|   Microchip Technology Inc.
|   PolarFire IBIS Model
[IBIS ver]   5.0
[File name]   polarfire_hsio_diff.ibs
[File Rev]   2.3
[Date]   Wed Nov 22 2023
[Source] Simulated Models ONLY.
   All data is based on Spice simulation. All performed at Microchip Technology Inc.
[Notes]   This IBIS file is for HSIO Differential standards.
   Please refer to polarfire_hsio_se.ibs for HSIO single ended Standards Configurations,
   and refer to polarfire_gpio_se.ibs and polarfire_gpio_diff.ibs for GPIO Configurations.
   The package parasitics of various package types are given.
   Uncomment the appropriate package before simulations.
   Revision History
   Rev 2.3: 22-Nov-2023
   - Added mixed mode receiver support:
   - Input buffers: HSTL12_18_ODT-OFF,HSTL12_15_ODT-OFF,HSTL12_135_ODT-OFF,
   HSTL135_18_ODT-OFF,HSTL135_15_ODT-OFF,HSTL15_18_ODT-OFF,
   HSUL12_18_ODT-OFF,HSUL12_18_ODT-60,HSUL12_18_ODT-120,HSUL12_18_ODT-240,
   HSUL12_15_ODT-OFF,HSUL12_15_ODT-60,HSUL12_15_ODT-120,HSUL12_15_ODT-240,
   HSUL12_135_ODT-OFF,HSUL12_135_ODT-60,HSUL12_135_ODT-120,HSUL12_135_ODT-240,
   POD12_18_ODT-OFF,POD12_15_ODT-OFF,POD12_135_ODT-OFF,SSTL135_18_ODT-OFF,
   SSTL135_15_ODT-OFF,SSTL15_18_ODT-OFF
   Rev 2.2: 20-Jun-2023
   - Added VCM-LOW configuration support for LVDS18,RSDS18,MINILVDS18,
   SUBLVDS18,PPDS18,SLVS18,HCSL18 receivers
   - Updated Vinl and Vinh values of LVDS18,SLVS18 receivers
   Rev 2.1: 14-Sep-2022
   - Added MPF050 device with RLC package data in [Package] section
   - Added LPDDR4 LVSTL11D I/O standard
   - Added RLC package type of FCG784N for MPF300T/TS device
   - Update RLC values of 200T-FCVG484 device package data
[Disclaimer] This information is for board design considerations.
   Simulation based V/I curves contained in this model file are
   considered preliminary until verified against bench
   measurements. Maximum currents may vary from part to part but
   should not exceed maximum I/V curves provided in this model file.
[Copyright]  (c) 2023, Microchip Technology Inc., All Rights Reserved.
| ADDITIONAL NOTES
| Warnings for ISSO Pullup, Pulldown currents being non-zero are expected.
| The naming conventions used in the signal_name/model_name are as follows:
| SLEW-#  - Slew setting,OFF or ON represented by #
| HYST-# and HYS-#  - Hysteresis setting,OFF or ON represented by #
| #mA   - Driver current strength, value represented by #
| #ohm   - Driver impedance mode, value represented by #
| ODT-# and OD-#   - Series on-die termination, impedance value represented by #
| C1   - Refers to Class-I driver models
| C2   - Refers to Class-II driver models
| #_I   - Refers to input models ,  model name represented by #
| #_O   - Refers to output models , model name represented by #
| VCML   - Refers to LOW Vcm setting
| VCMM   - Refers to MID Vcm setting
| IBIS MODEL CHECKLIST
| Microchip Technology Inc. is dedicated to releasing quality IBIS models to customers.
| The following items have been
| verified for this IBIS model before release:
| 1)  Checked IBIS model by the golden parser ibischk5 [Complete]
| 2)  Ensured no errors reported by golden parser
|   for the IBIS model [Complete]
| 3)  Defined Vinl and Vinh for receivers [Complete]
| 4)  Defined Standard Load and Vmeas values for drivers [Complete]
| 5)  Defined overshoots for drivers and receivers [NA]
| 6)  Validated Ramp Values[]
| 7)  Defined V-T Tables for all output drivers [Complete]
| 8)  Validated [Diff Pins] [Complete]
| 9)  Verified Package Parasitics [Complete]
| 10) Defined Standard Load Parameters and Specifications
|   for waveforms [Complete]
| 11) Defined and Validate Pin mappings [Complete]
| 12) Verified C_comp_pullup and C_comp_pulldown Values []
| 13) Visually Inspected I-V Curves and V-T Tables  [Complete]
| 14) Presented Typ/Min/Max Values in the correct order for
|   all tables and parameters [Complete]
| 15) Simulated all output models with standard load and
|   switching through Vmeas [Complete]
| 16) Simulated all receiver models  [Complete]
| 17) Validated Models selectors. [NA]
| 18) Visually inspected Spice and IBIS correlation for
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[Component]   PolarFire
[Manufacturer]   Microchip Technology Inc.
[Package]
|   typ   min   max
|MPF050T/TL/TLS/TS
|R_pkg   0.424   NA   NA   | MPF050T/TL/TLS/TS-FCSG325
|L_pkg   2.847nH   NA   NA   | MPF050T/TL/TLS/TS-FCSG325
|C_pkg   1.075pF   NA   NA   | MPF050T/TL/TLS/TS-FCSG325
|R_pkg   0.726   NA   NA   | MPF050T/TL/TLS/TS-FCVG484
|L_pkg   5.270nH   NA   NA   | MPF050T/TL/TLS/TS-FCVG484
|C_pkg   1.827pF   NA   NA   | MPF050T/TL/TLS/TS-FCVG484
|MPF100T/TL/TLS/TS
|R_pkg   0.300925   NA   NA   | MPF100T/TL/TLS/TS-FCSG325
|L_pkg   2.47653nH   NA   NA   | MPF100T/TL/TLS/TS-FCSG325
|C_pkg   1.00755pF   NA   NA   | MPF100T/TL/TLS/TS-FCSG325
|R_pkg   0.873007   NA   NA   | MPF100T/TL/TLS/TS-FCG484
|L_pkg   5.7244nH   NA   NA   | MPF100T/TL/TLS/TS-FCG484
|C_pkg   2.04208pF   NA   NA   | MPF100T/TL/TLS/TS-FCG484
|R_pkg   0.61   NA   NA   | MPF100T/TL/TLS/TS-FCVG484
|L_pkg   4.49536nH   NA   NA   | MPF100T/TL/TLS/TS-FCVG484
|C_pkg   1.77743pF   NA   NA   | MPF100T/TL/TLS/TS-FCVG484
|MPF200T/TL/TLS/TS
|R_pkg   0.570552   NA   NA   | MPF200T/TL/TLS/TS-FCSG325
|L_pkg   4.57321nH   NA   NA   | MPF200T/TL/TLS/TS-FCSG325
|C_pkg   1.39793pF   NA   NA   | MPF200T/TL/TLS/TS-FCSG325
|R_pkg   0.813737   NA   NA   | MPF200T/TL/TLS/TS-FCG484
|L_pkg   5.39433nH   NA   NA   | MPF200T/TL/TLS/TS-FCG484
|C_pkg   1.90867pF   NA   NA   | MPF200T/TL/TLS/TS-FCG484
|R_pkg   0.592554   NA   NA   | MPF200T/TL/TLS/TS-FCVG484
|L_pkg   4.00867nH   NA   NA   | MPF200T/TL/TLS/TS-FCVG484
|C_pkg   1.56354pF   NA   NA   | MPF200T/TL/TLS/TS-FCVG484
|R_pkg   0.39999   NA   NA   | MPF200T/TL/TLS/TS-FCSG536
|L_pkg   3.20603nH   NA   NA   | MPF200T/TL/TLS/TS-FCSG536
|C_pkg   1.22995pF   NA   NA   | MPF200T/TL/TLS/TS-FCSG536
|R_pkg   1.32073   NA   NA   | MPF200T/TL/TLS/TS-FCG784
|L_pkg   8.15293nH   NA   NA   | MPF200T/TL/TLS/TS-FCG784
|C_pkg   2.72193pF   NA   NA   | MPF200T/TL/TLS/TS-FCG784
|MPF300T/TL/TLS/TS
|R_pkg   0.713491   NA   NA   | MPF300T/TL/TLS/TS-FCG484
|L_pkg   4.77635nH   NA   NA   | MPF300T/TL/TLS/TS-FCG484
|C_pkg   1.82577pF   NA   NA   | MPF300T/TL/TLS/TS-FCG484
|R_pkg   0.493927   NA   NA   | MPF300T/TL/TLS/TS-FCVG484
|L_pkg   3.29806nH   NA   NA   | MPF300T/TL/TLS/TS-FCVG484
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R_pkg   1.65645   NA   NA   | MPF300T/TL/TLS/TS-FCG1152
L_pkg   9.92288nH   NA   NA   | MPF300T/TL/TLS/TS-FCG1152
C_pkg   3.06321pF   NA   NA   | MPF300T/TL/TLS/TS-FCG1152
|MPF500T/TL/TLS/TS
|R_pkg   0.914871   NA   NA   | MPF500T/TL/TLS/TS-FCG784
|L_pkg   5.88658nH   NA   NA   | MPF500T/TL/TLS/TS-FCG784
|C_pkg   2.0993pF   NA   NA   | MPF500T/TL/TLS/TS-FCG784
|R_pkg   1.46382   NA   NA   | MPF500T/TL/TLS/TS-FCG1152
|L_pkg   9.31721nH   NA   NA   | MPF500T/TL/TLS/TS-FCG1152
|C_pkg   2.98723pF   NA   NA   | MPF500T/TL/TLS/TS-FCG1152
| End Header
| The PIN numbers given below are examples. They do not correspond to
| device pin numbers.
[Pin]   signal_name   model_name   R_pin   L_pin   C_pin
1N   SSTL18D_C1_60ohm_SLEW-OFF_N_O   SSTL18_C1_60ohm_SLEW-OFF_HSIO_O
1P   SSTL18D_C1_60ohm_SLEW-OFF_P_O   SSTL18_C1_60ohm_SLEW-OFF_HSIO_O
2N   SSTL18D_C1_80ohm_SLEW-OFF_N_O   SSTL18_C1_80ohm_SLEW-OFF_HSIO_O
2P   SSTL18D_C1_80ohm_SLEW-OFF_P_O   SSTL18_C1_80ohm_SLEW-OFF_HSIO_O
3N   SSTL18D_C1_48ohm_SLEW-OFF_N_O   SSTL18_C1_48ohm_SLEW-OFF_HSIO_O
3P   SSTL18D_C1_48ohm_SLEW-OFF_P_O   SSTL18_C1_48ohm_SLEW-OFF_HSIO_O
4N   SSTL18D_C1_40ohm_SLEW-OFF_N_O   SSTL18_C1_40ohm_SLEW-OFF_HSIO_O
4P   SSTL18D_C1_40ohm_SLEW-OFF_P_O   SSTL18_C1_40ohm_SLEW-OFF_HSIO_O
5N   SSTL18D_C2_40ohm_SLEW-OFF_N_O   SSTL18_C2_40ohm_SLEW-OFF_HSIO_O
5P   SSTL18D_C2_40ohm_SLEW-OFF_P_O   SSTL18_C2_40ohm_SLEW-OFF_HSIO_O
6N   SSTL18D_C2_48ohm_SLEW-OFF_N_O   SSTL18_C2_48ohm_SLEW-OFF_HSIO_O
6P   SSTL18D_C2_48ohm_SLEW-OFF_P_O   SSTL18_C2_48ohm_SLEW-OFF_HSIO_O
7N   SSTL18D_C2_34ohm_SLEW-OFF_N_O   SSTL18_C2_34ohm_SLEW-OFF_HSIO_O
7P   SSTL18D_C2_34ohm_SLEW-OFF_P_O   SSTL18_C2_34ohm_SLEW-OFF_HSIO_O
8N   SSTL18D_C2_30ohm_SLEW-OFF_N_O   SSTL18_C2_30ohm_SLEW-OFF_HSIO_O
8P   SSTL18D_C2_30ohm_SLEW-OFF_P_O   SSTL18_C2_30ohm_SLEW-OFF_HSIO_O
9N   SSTL15D_C1_40ohm_SLEW-OFF_N_O   SSTL15_C1_40ohm_SLEW-OFF_HSIO_O
9P   SSTL15D_C1_40ohm_SLEW-OFF_P_O   SSTL15_C1_40ohm_SLEW-OFF_HSIO_O
10N   SSTL15D_C1_48ohm_SLEW-OFF_N_O   SSTL15_C1_48ohm_SLEW-OFF_HSIO_O
10P   SSTL15D_C1_48ohm_SLEW-OFF_P_O   SSTL15_C1_48ohm_SLEW-OFF_HSIO_O
11N   SSTL15D_C2_34ohm_SLEW-OFF_N_O   SSTL15_C2_34ohm_SLEW-OFF_HSIO_O
11P   SSTL15D_C2_34ohm_SLEW-OFF_P_O   SSTL15_C2_34ohm_SLEW-OFF_HSIO_O
12N   SSTL15D_C2_30ohm_SLEW-OFF_N_O   SSTL15_C2_30ohm_SLEW-OFF_HSIO_O
12P   SSTL15D_C2_30ohm_SLEW-OFF_P_O   SSTL15_C2_30ohm_SLEW-OFF_HSIO_O
13N   SSTL15D_C2_27ohm_SLEW-OFF_N_O   SSTL15_C2_27ohm_SLEW-OFF_HSIO_O
13P   SSTL15D_C2_27ohm_SLEW-OFF_P_O   SSTL15_C2_27ohm_SLEW-OFF_HSIO_O
14N   SSTL135D_C1_40ohm_SLEW-OFF_N_O   SSTL135_C1_40ohm_SLEW-OFF_HSIO_O
14P   SSTL135D_C1_40ohm_SLEW-OFF_P_O   SSTL135_C1_40ohm_SLEW-OFF_HSIO_O
15N   SSTL135D_C1_48ohm_SLEW-OFF_N_O   SSTL135_C1_48ohm_SLEW-OFF_HSIO_O
15P   SSTL135D_C1_48ohm_SLEW-OFF_P_O   SSTL135_C1_48ohm_SLEW-OFF_HSIO_O
16N   SSTL135D_C2_34ohm_SLEW-OFF_N_O   SSTL135_C2_34ohm_SLEW-OFF_HSIO_O
16P   SSTL135D_C2_34ohm_SLEW-OFF_P_O   SSTL135_C2_34ohm_SLEW-OFF_HSIO_O
17N   SSTL135D_C2_30ohm_SLEW-OFF_N_O   SSTL135_C2_30ohm_SLEW-OFF_HSIO_O
17P   SSTL135D_C2_30ohm_SLEW-OFF_P_O   SSTL135_C2_30ohm_SLEW-OFF_HSIO_O
18N   SSTL135D_C2_27ohm_SLEW-OFF_N_O   SSTL135_C2_27ohm_SLEW-OFF_HSIO_O
18P   SSTL135D_C2_27ohm_SLEW-OFF_P_O   SSTL135_C2_27ohm_SLEW-OFF_HSIO_O
19N   HSUL18D_C1_55ohm_SLEW-OFF_N_O   HSUL18_C1_55ohm_SLEW-OFF_HSIO_O
19P   HSUL18D_C1_55ohm_SLEW-OFF_P_O   HSUL18_C1_55ohm_SLEW-OFF_HSIO_O
20N   HSUL18D_C1_60ohm_SLEW-OFF_N_O   HSUL18_C1_60ohm_SLEW-OFF_HSIO_O
20P   HSUL18D_C1_60ohm_SLEW-OFF_P_O   HSUL18_C1_60ohm_SLEW-OFF_HSIO_O
21N   HSUL18D_C1_40ohm_SLEW-OFF_N_O   HSUL18_C1_40ohm_SLEW-OFF_HSIO_O
21P   HSUL18D_C1_40ohm_SLEW-OFF_P_O   HSUL18_C1_40ohm_SLEW-OFF_HSIO_O
22N   HSUL18D_C1_34ohm_SLEW-OFF_N_O   HSUL18_C1_34ohm_SLEW-OFF_HSIO_O
22P   HSUL18D_C1_34ohm_SLEW-OFF_P_O   HSUL18_C1_34ohm_SLEW-OFF_HSIO_O
23N   HSUL18D_C2_25ohm_SLEW-OFF_N_O   HSUL18_C2_25ohm_SLEW-OFF_HSIO_O
23P   HSUL18D_C2_25ohm_SLEW-OFF_P_O   HSUL18_C2_25ohm_SLEW-OFF_HSIO_O
24N   HSUL18D_C2_30ohm_SLEW-OFF_N_O   HSUL18_C2_30ohm_SLEW-OFF_HSIO_O
24P   HSUL18D_C2_30ohm_SLEW-OFF_P_O   HSUL18_C2_30ohm_SLEW-OFF_HSIO_O
25N   HSUL18D_C2_27ohm_SLEW-OFF_N_O   HSUL18_C2_27ohm_SLEW-OFF_HSIO_O
25P   HSUL18D_C2_27ohm_SLEW-OFF_P_O   HSUL18_C2_27ohm_SLEW-OFF_HSIO_O
26N   HSUL18D_C2_22ohm_SLEW-OFF_N_O   HSUL18_C2_22ohm_SLEW-OFF_HSIO_O
26P   HSUL18D_C2_22ohm_SLEW-OFF_P_O   HSUL18_C2_22ohm_SLEW-OFF_HSIO_O
27N   HSTL15D_C1_50ohm_SLEW-OFF_N_O   HSTL15_C1_50ohm_SLEW-OFF_HSIO_O
27P   HSTL15D_C1_50ohm_SLEW-OFF_P_O   HSTL15_C1_50ohm_SLEW-OFF_HSIO_O
28N   HSTL15D_C1_60ohm_SLEW-OFF_N_O   HSTL15_C1_60ohm_SLEW-OFF_HSIO_O
28P   HSTL15D_C1_60ohm_SLEW-OFF_P_O   HSTL15_C1_60ohm_SLEW-OFF_HSIO_O
29N   HSTL15D_C1_40ohm_SLEW-OFF_N_O   HSTL15_C1_40ohm_SLEW-OFF_HSIO_O
29P   HSTL15D_C1_40ohm_SLEW-OFF_P_O   HSTL15_C1_40ohm_SLEW-OFF_HSIO_O
30N   HSTL15D_C1_34ohm_SLEW-OFF_N_O   HSTL15_C1_34ohm_SLEW-OFF_HSIO_O
30P   HSTL15D_C1_34ohm_SLEW-OFF_P_O   HSTL15_C1_34ohm_SLEW-OFF_HSIO_O
31N   HSTL15D_C2_25ohm_SLEW-OFF_N_O   HSTL15_C2_25ohm_SLEW-OFF_HSIO_O
31P   HSTL15D_C2_25ohm_SLEW-OFF_P_O   HSTL15_C2_25ohm_SLEW-OFF_HSIO_O
32N   HSTL15D_C2_30ohm_SLEW-OFF_N_O   HSTL15_C2_30ohm_SLEW-OFF_HSIO_O
32P   HSTL15D_C2_30ohm_SLEW-OFF_P_O   HSTL15_C2_30ohm_SLEW-OFF_HSIO_O
33N   HSTL15D_C2_27ohm_SLEW-OFF_N_O   HSTL15_C2_27ohm_SLEW-OFF_HSIO_O
33P   HSTL15D_C2_27ohm_SLEW-OFF_P_O   HSTL15_C2_27ohm_SLEW-OFF_HSIO_O
34N   HSTL15D_C2_22ohm_SLEW-OFF_N_O   HSTL15_C2_22ohm_SLEW-OFF_HSIO_O
34P   HSTL15D_C2_22ohm_SLEW-OFF_P_O   HSTL15_C2_22ohm_SLEW-OFF_HSIO_O
35N   HSTL135D_C1_50ohm_SLEW-OFF_N_O   HSTL135_C1_50ohm_SLEW-OFF_HSIO_O
35P   HSTL135D_C1_50ohm_SLEW-OFF_P_O   HSTL135_C1_50ohm_SLEW-OFF_HSIO_O
36N   HSTL135D_C1_60ohm_SLEW-OFF_N_O   HSTL135_C1_60ohm_SLEW-OFF_HSIO_O
36P   HSTL135D_C1_60ohm_SLEW-OFF_P_O   HSTL135_C1_60ohm_SLEW-OFF_HSIO_O
37N   HSTL135D_C1_40ohm_SLEW-OFF_N_O   HSTL135_C1_40ohm_SLEW-OFF_HSIO_O
37P   HSTL135D_C1_40ohm_SLEW-OFF_P_O   HSTL135_C1_40ohm_SLEW-OFF_HSIO_O
38N   HSTL135D_C1_34ohm_SLEW-OFF_N_O   HSTL135_C1_34ohm_SLEW-OFF_HSIO_O
38P   HSTL135D_C1_34ohm_SLEW-OFF_P_O   HSTL135_C1_34ohm_SLEW-OFF_HSIO_O
39N   HSTL135D_C2_25ohm_SLEW-OFF_N_O   HSTL135_C2_25ohm_SLEW-OFF_HSIO_O
39P   HSTL135D_C2_25ohm_SLEW-OFF_P_O   HSTL135_C2_25ohm_SLEW-OFF_HSIO_O
40N   HSTL135D_C2_30ohm_SLEW-OFF_N_O   HSTL135_C2_30ohm_SLEW-OFF_HSIO_O
40P   HSTL135D_C2_30ohm_SLEW-OFF_P_O   HSTL135_C2_30ohm_SLEW-OFF_HSIO_O
41N   HSTL135D_C2_27ohm_SLEW-OFF_N_O   HSTL135_C2_27ohm_SLEW-OFF_HSIO_O
41P   HSTL135D_C2_27ohm_SLEW-OFF_P_O   HSTL135_C2_27ohm_SLEW-OFF_HSIO_O
42N   HSTL135D_C2_22ohm_SLEW-OFF_N_O   HSTL135_C2_22ohm_SLEW-OFF_HSIO_O
42P   HSTL135D_C2_22ohm_SLEW-OFF_P_O   HSTL135_C2_22ohm_SLEW-OFF_HSIO_O
43N   HSUL12D_40ohm_SLEW-OFF_N_O   HSUL12_40ohm_SLEW-OFF_HSIO_O
43P   HSUL12D_40ohm_SLEW-OFF_P_O   HSUL12_40ohm_SLEW-OFF_HSIO_O
44N   HSUL12D_120ohm_SLEW-OFF_N_O   HSUL12_120ohm_SLEW-OFF_HSIO_O
44P   HSUL12D_120ohm_SLEW-OFF_P_O   HSUL12_120ohm_SLEW-OFF_HSIO_O
45N   HSUL12D_80ohm_SLEW-OFF_N_O   HSUL12_80ohm_SLEW-OFF_HSIO_O
45P   HSUL12D_80ohm_SLEW-OFF_P_O   HSUL12_80ohm_SLEW-OFF_HSIO_O
46N   HSUL12D_60ohm_SLEW-OFF_N_O   HSUL12_60ohm_SLEW-OFF_HSIO_O
46P   HSUL12D_60ohm_SLEW-OFF_P_O   HSUL12_60ohm_SLEW-OFF_HSIO_O
47N   HSUL12D_48ohm_SLEW-OFF_N_O   HSUL12_48ohm_SLEW-OFF_HSIO_O
47P   HSUL12D_48ohm_SLEW-OFF_P_O   HSUL12_48ohm_SLEW-OFF_HSIO_O
48N   HSUL12D_34ohm_SLEW-OFF_N_O   HSUL12_34ohm_SLEW-OFF_HSIO_O
48P   HSUL12D_34ohm_SLEW-OFF_P_O   HSUL12_34ohm_SLEW-OFF_HSIO_O
49N   POD12D_C1_48ohm_SLEW-OFF_N_O   POD12_C1_48ohm_SLEW-OFF_HSIO_O
49P   POD12D_C1_48ohm_SLEW-OFF_P_O   POD12_C1_48ohm_SLEW-OFF_HSIO_O
50N   POD12D_C1_60ohm_SLEW-OFF_N_O   POD12_C1_60ohm_SLEW-OFF_HSIO_O
50P   POD12D_C1_60ohm_SLEW-OFF_P_O   POD12_C1_60ohm_SLEW-OFF_HSIO_O
51N   POD12D_C1_40ohm_SLEW-OFF_N_O   POD12_C1_40ohm_SLEW-OFF_HSIO_O
51P   POD12D_C1_40ohm_SLEW-OFF_P_O   POD12_C1_40ohm_SLEW-OFF_HSIO_O
52N   POD12D_C2_34ohm_SLEW-OFF_N_O   POD12_C2_34ohm_SLEW-OFF_HSIO_O
52P   POD12D_C2_34ohm_SLEW-OFF_P_O   POD12_C2_34ohm_SLEW-OFF_HSIO_O
53N   POD12D_C2_30ohm_SLEW-OFF_N_O   POD12_C2_30ohm_SLEW-OFF_HSIO_O
53P   POD12D_C2_30ohm_SLEW-OFF_P_O   POD12_C2_30ohm_SLEW-OFF_HSIO_O
54N   POD12D_C2_27ohm_SLEW-OFF_N_O   POD12_C2_27ohm_SLEW-OFF_HSIO_O
54P   POD12D_C2_27ohm_SLEW-OFF_P_O   POD12_C2_27ohm_SLEW-OFF_HSIO_O
55N   HSTL12D_C1_50ohm_SLEW-OFF_N_O   HSTL12_C1_50ohm_SLEW-OFF_HSIO_O
55P   HSTL12D_C1_50ohm_SLEW-OFF_P_O   HSTL12_C1_50ohm_SLEW-OFF_HSIO_O
56N   HSTL12D_C2_25ohm_SLEW-OFF_N_O   HSTL12_C2_25ohm_SLEW-OFF_HSIO_O
56P   HSTL12D_C2_25ohm_SLEW-OFF_P_O   HSTL12_C2_25ohm_SLEW-OFF_HSIO_O
57N   LVCMOS18D_8mA_SLEW-OFF_N_O   LVCMOS18_8mA_SLEW-OFF_HSIO_O
57P   LVCMOS18D_8mA_SLEW-OFF_P_O   LVCMOS18_8mA_SLEW-OFF_HSIO_O
58N   LVCMOS18D_2mA_SLEW-OFF_N_O   LVCMOS18_2mA_SLEW-OFF_HSIO_O
58P   LVCMOS18D_2mA_SLEW-OFF_P_O   LVCMOS18_2mA_SLEW-OFF_HSIO_O
59N   LVCMOS18D_4mA_SLEW-OFF_N_O   LVCMOS18_4mA_SLEW-OFF_HSIO_O
59P   LVCMOS18D_4mA_SLEW-OFF_P_O   LVCMOS18_4mA_SLEW-OFF_HSIO_O
60N   LVCMOS18D_6mA_SLEW-OFF_N_O   LVCMOS18_6mA_SLEW-OFF_HSIO_O
60P   LVCMOS18D_6mA_SLEW-OFF_P_O   LVCMOS18_6mA_SLEW-OFF_HSIO_O
61N   LVCMOS18D_10mA_SLEW-OFF_N_O   LVCMOS18_10mA_SLEW-OFF_HSIO_O
61P   LVCMOS18D_10mA_SLEW-OFF_P_O   LVCMOS18_10mA_SLEW-OFF_HSIO_O
62N   LVCMOS18D_12mA_SLEW-OFF_N_O   LVCMOS18_12mA_SLEW-OFF_HSIO_O
62P   LVCMOS18D_12mA_SLEW-OFF_P_O   LVCMOS18_12mA_SLEW-OFF_HSIO_O
63N   LVCMOS15D_8mA_SLEW-OFF_N_O   LVCMOS15_8mA_SLEW-OFF_HSIO_O
63P   LVCMOS15D_8mA_SLEW-OFF_P_O   LVCMOS15_8mA_SLEW-OFF_HSIO_O
64N   LVCMOS15D_2mA_SLEW-OFF_N_O   LVCMOS15_2mA_SLEW-OFF_HSIO_O
64P   LVCMOS15D_2mA_SLEW-OFF_P_O   LVCMOS15_2mA_SLEW-OFF_HSIO_O
65N   LVCMOS15D_4mA_SLEW-OFF_N_O   LVCMOS15_4mA_SLEW-OFF_HSIO_O
65P   LVCMOS15D_4mA_SLEW-OFF_P_O   LVCMOS15_4mA_SLEW-OFF_HSIO_O
66N   LVCMOS15D_6mA_SLEW-OFF_N_O   LVCMOS15_6mA_SLEW-OFF_HSIO_O
66P   LVCMOS15D_6mA_SLEW-OFF_P_O   LVCMOS15_6mA_SLEW-OFF_HSIO_O
67N   LVCMOS15D_10mA_SLEW-OFF_N_O   LVCMOS15_10mA_SLEW-OFF_HSIO_O
67P   LVCMOS15D_10mA_SLEW-OFF_P_O   LVCMOS15_10mA_SLEW-OFF_HSIO_O
68N   LVCMOS12D_8mA_SLEW-OFF_N_O   LVCMOS12_8mA_SLEW-OFF_HSIO_O
68P   LVCMOS12D_8mA_SLEW-OFF_P_O   LVCMOS12_8mA_SLEW-OFF_HSIO_O
69N   LVCMOS12D_2mA_SLEW-OFF_N_O   LVCMOS12_2mA_SLEW-OFF_HSIO_O
69P   LVCMOS12D_2mA_SLEW-OFF_P_O   LVCMOS12_2mA_SLEW-OFF_HSIO_O
70N   LVCMOS12D_4mA_SLEW-OFF_N_O   LVCMOS12_4mA_SLEW-OFF_HSIO_O
70P   LVCMOS12D_4mA_SLEW-OFF_P_O   LVCMOS12_4mA_SLEW-OFF_HSIO_O
71N   LVCMOS12D_6mA_SLEW-OFF_N_O   LVCMOS12_6mA_SLEW-OFF_HSIO_O
71P   LVCMOS12D_6mA_SLEW-OFF_P_O   LVCMOS12_6mA_SLEW-OFF_HSIO_O
72N   LVCMOS12D_10mA_SLEW-OFF_N_O   LVCMOS12_10mA_SLEW-OFF_HSIO_O
72P   LVCMOS12D_10mA_SLEW-OFF_P_O   LVCMOS12_10mA_SLEW-OFF_HSIO_O
73N   SSTL18D_ODT-OFF_HYST-OFF_N_I   SSTL18_ODT-OFF_HYST-OFF_HSIO_I
73P   SSTL18D_ODT-OFF_HYST-OFF_P_I   SSTL18_ODT-OFF_HYST-OFF_HSIO_I
74N   SSTL18D_ODT-50_HYST-OFF_N_I   SSTL18_ODT-50_HYST-OFF_HSIO_I
74P   SSTL18D_ODT-50_HYST-OFF_P_I   SSTL18_ODT-50_HYST-OFF_HSIO_I
75N   SSTL18D_ODT-150_HYST-OFF_N_I   SSTL18_ODT-150_HYST-OFF_HSIO_I
75P   SSTL18D_ODT-150_HYST-OFF_P_I   SSTL18_ODT-150_HYST-OFF_HSIO_I
76N   SSTL18D_ODT-75_HYST-OFF_N_I   SSTL18_ODT-75_HYST-OFF_HSIO_I
76P   SSTL18D_ODT-75_HYST-OFF_P_I   SSTL18_ODT-75_HYST-OFF_HSIO_I
77N   SSTL15D_ODT-OFF_HYST-OFF_N_I   SSTL15_ODT-OFF_HYST-OFF_HSIO_I
77P   SSTL15D_ODT-OFF_HYST-OFF_P_I   SSTL15_ODT-OFF_HYST-OFF_HSIO_I
78N   SSTL15D_ODT-60_HYST-OFF_N_I   SSTL15_ODT-60_HYST-OFF_HSIO_I
78P   SSTL15D_ODT-60_HYST-OFF_P_I   SSTL15_ODT-60_HYST-OFF_HSIO_I
79N   SSTL15D_ODT-120_HYST-OFF_N_I   SSTL15_ODT-120_HYST-OFF_HSIO_I
79P   SSTL15D_ODT-120_HYST-OFF_P_I   SSTL15_ODT-120_HYST-OFF_HSIO_I
80N   SSTL15D_ODT-40_HYST-OFF_N_I   SSTL15_ODT-40_HYST-OFF_HSIO_I
80P   SSTL15D_ODT-40_HYST-OFF_P_I   SSTL15_ODT-40_HYST-OFF_HSIO_I
81N   SSTL15D_ODT-30_HYST-OFF_N_I   SSTL15_ODT-30_HYST-OFF_HSIO_I
81P   SSTL15D_ODT-30_HYST-OFF_P_I   SSTL15_ODT-30_HYST-OFF_HSIO_I
82N   SSTL15D_ODT-20_HYST-OFF_N_I   SSTL15_ODT-20_HYST-OFF_HSIO_I
82P   SSTL15D_ODT-20_HYST-OFF_P_I   SSTL15_ODT-20_HYST-OFF_HSIO_I
83N   SSTL135D_ODT-OFF_HYST-OFF_N_I   SSTL135_ODT-OFF_HYST-OFF_HSIO_I
83P   SSTL135D_ODT-OFF_HYST-OFF_P_I   SSTL135_ODT-OFF_HYST-OFF_HSIO_I
84N   SSTL135D_ODT-60_HYST-OFF_N_I   SSTL135_ODT-60_HYST-OFF_HSIO_I
84P   SSTL135D_ODT-60_HYST-OFF_P_I   SSTL135_ODT-60_HYST-OFF_HSIO_I
85N   SSTL135D_ODT-120_HYST-OFF_N_I   SSTL135_ODT-120_HYST-OFF_HSIO_I
85P   SSTL135D_ODT-120_HYST-OFF_P_I   SSTL135_ODT-120_HYST-OFF_HSIO_I
86N   SSTL135D_ODT-40_HYST-OFF_N_I   SSTL135_ODT-40_HYST-OFF_HSIO_I
86P   SSTL135D_ODT-40_HYST-OFF_P_I   SSTL135_ODT-40_HYST-OFF_HSIO_I
87N   SSTL135D_ODT-30_HYST-OFF_N_I   SSTL135_ODT-30_HYST-OFF_HSIO_I
87P   SSTL135D_ODT-30_HYST-OFF_P_I   SSTL135_ODT-30_HYST-OFF_HSIO_I
88N   SSTL135D_ODT-20_HYST-OFF_N_I   SSTL135_ODT-20_HYST-OFF_HSIO_I
88P   SSTL135D_ODT-20_HYST-OFF_P_I   SSTL135_ODT-20_HYST-OFF_HSIO_I
89N   HSUL18D_ODT-OFF_HYST-OFF_N_I   HSUL18_ODT-OFF_HYST-OFF_HSIO_I
89P   HSUL18D_ODT-OFF_HYST-OFF_P_I   HSUL18_ODT-OFF_HYST-OFF_HSIO_I
90N   HSUL18D_ODT-50_HYST-OFF_N_I   HSUL18_ODT-50_HYST-OFF_HSIO_I
90P   HSUL18D_ODT-50_HYST-OFF_P_I   HSUL18_ODT-50_HYST-OFF_HSIO_I
91N   HSTL15D_ODT-OFF_HYST-OFF_N_I   HSTL15_ODT-OFF_HYST-OFF_HSIO_I
91P   HSTL15D_ODT-OFF_HYST-OFF_P_I   HSTL15_ODT-OFF_HYST-OFF_HSIO_I
92N   HSTL15D_ODT-50_HYST-OFF_N_I   HSTL15_ODT-50_HYST-OFF_HSIO_I
92P   HSTL15D_ODT-50_HYST-OFF_P_I   HSTL15_ODT-50_HYST-OFF_HSIO_I
93N   HSTL135D_ODT-OFF_HYST-OFF_N_I   HSTL135_ODT-OFF_HYST-OFF_HSIO_I
93P   HSTL135D_ODT-OFF_HYST-OFF_P_I   HSTL135_ODT-OFF_HYST-OFF_HSIO_I
94N   HSTL135D_ODT-50_HYST-OFF_N_I   HSTL135_ODT-50_HYST-OFF_HSIO_I
94P   HSTL135D_ODT-50_HYST-OFF_P_I   HSTL135_ODT-50_HYST-OFF_HSIO_I
95N   HSUL12D_ODT-OFF_HYST-OFF_N_I   HSUL12_ODT-OFF_HYST-OFF_HSIO_I
95P   HSUL12D_ODT-OFF_HYST-OFF_P_I   HSUL12_ODT-OFF_HYST-OFF_HSIO_I
96N   HSUL12D_ODT-60_HYST-OFF_N_I   HSUL12_ODT-60_HYST-OFF_HSIO_I
96P   HSUL12D_ODT-60_HYST-OFF_P_I   HSUL12_ODT-60_HYST-OFF_HSIO_I
97N   HSUL12D_ODT-240_HYST-OFF_N_I   HSUL12_ODT-240_HYST-OFF_HSIO_I
97P   HSUL12D_ODT-240_HYST-OFF_P_I   HSUL12_ODT-240_HYST-OFF_HSIO_I
98N   HSUL12D_ODT-120_HYST-OFF_N_I   HSUL12_ODT-120_HYST-OFF_HSIO_I
98P   HSUL12D_ODT-120_HYST-OFF_P_I   HSUL12_ODT-120_HYST-OFF_HSIO_I
99N   POD12D_ODT-OFF_HYST-OFF_N_I   POD12_ODT-OFF_HYST-OFF_HSIO_I
99P   POD12D_ODT-OFF_HYST-OFF_P_I   POD12_ODT-OFF_HYST-OFF_HSIO_I
100N   POD12D_ODT-60_HYST-OFF_N_I   POD12_ODT-60_HYST-OFF_HSIO_I
100P   POD12D_ODT-60_HYST-OFF_P_I   POD12_ODT-60_HYST-OFF_HSIO_I
101N   POD12D_ODT-240_HYST-OFF_N_I   POD12_ODT-240_HYST-OFF_HSIO_I
101P   POD12D_ODT-240_HYST-OFF_P_I   POD12_ODT-240_HYST-OFF_HSIO_I
102N   POD12D_ODT-120_HYST-OFF_N_I   POD12_ODT-120_HYST-OFF_HSIO_I
102P   POD12D_ODT-120_HYST-OFF_P_I   POD12_ODT-120_HYST-OFF_HSIO_I
103N   POD12D_ODT-80_HYST-OFF_N_I   POD12_ODT-80_HYST-OFF_HSIO_I
103P   POD12D_ODT-80_HYST-OFF_P_I   POD12_ODT-80_HYST-OFF_HSIO_I
104N   POD12D_ODT-48_HYST-OFF_N_I   POD12_ODT-48_HYST-OFF_HSIO_I
104P   POD12D_ODT-48_HYST-OFF_P_I   POD12_ODT-48_HYST-OFF_HSIO_I
105N   POD12D_ODT-40_HYST-OFF_N_I   POD12_ODT-40_HYST-OFF_HSIO_I
105P   POD12D_ODT-40_HYST-OFF_P_I   POD12_ODT-40_HYST-OFF_HSIO_I
106N   POD12D_ODT-34_HYST-OFF_N_I   POD12_ODT-34_HYST-OFF_HSIO_I
106P   POD12D_ODT-34_HYST-OFF_P_I   POD12_ODT-34_HYST-OFF_HSIO_I
107N   HSTL12D_ODT-OFF_HYST-OFF_N_I   HSTL12_ODT-OFF_HYST-OFF_HSIO_I
107P   HSTL12D_ODT-OFF_HYST-OFF_P_I   HSTL12_ODT-OFF_HYST-OFF_HSIO_I
108N   HSTL12D_ODT-50_HYST-OFF_N_I   HSTL12_ODT-50_HYST-OFF_HSIO_I
108P   HSTL12D_ODT-50_HYST-OFF_P_I   HSTL12_ODT-50_HYST-OFF_HSIO_I
109N   LVDS18_ODT-OFF_HYST-OFF_N_I   LVDS18_ODT-OFF_HYST-OFF_HSIO_I
109P   LVDS18_ODT-OFF_HYST-OFF_P_I   LVDS18_ODT-OFF_HYST-OFF_HSIO_I
110N   RSDS18_ODT-OFF_HYST-OFF_N_I   RSDS18_ODT-OFF_HYST-OFF_HSIO_I
110P   RSDS18_ODT-OFF_HYST-OFF_P_I   RSDS18_ODT-OFF_HYST-OFF_HSIO_I
111N   MINILVDS18_ODT-OFF_HYST-OFF_N_I   MINILVDS18_ODT-OFF_HYST-OFF_HSIO_I
111P   MINILVDS18_ODT-OFF_HYST-OFF_P_I   MINILVDS18_ODT-OFF_HYST-OFF_HSIO_I
112N   SUBLVDS18_ODT-OFF_HYST-OFF_N_I   SUBLVDS18_ODT-OFF_HYST-OFF_HSIO_I
112P   SUBLVDS18_ODT-OFF_HYST-OFF_P_I   SUBLVDS18_ODT-OFF_HYST-OFF_HSIO_I
113N   PPDS18_ODT-OFF_HYST-OFF_N_I   PPDS18_ODT-OFF_HYST-OFF_HSIO_I
113P   PPDS18_ODT-OFF_HYST-OFF_P_I   PPDS18_ODT-OFF_HYST-OFF_HSIO_I
114N   LCMDS18_ODT-OFF_HYST-OFF_N_I   LCMDS18_ODT-OFF_HYST-OFF_HSIO_I
114P   LCMDS18_ODT-OFF_HYST-OFF_P_I   LCMDS18_ODT-OFF_HYST-OFF_HSIO_I
115N   SLVS18_ODT-OFF_HYST-OFF_N_I   SLVS18_ODT-OFF_HYST-OFF_N_HSIO_I
115P   SLVS18_ODT-OFF_HYST-OFF_P_I   SLVS18_ODT-OFF_HYST-OFF_P_HSIO_I
116N   HCSL18_ODT-OFF_HYST-OFF_N_I   HCSL18_ODT-OFF_HYST-OFF_HSIO_I
116P   HCSL18_ODT-OFF_HYST-OFF_P_I   HCSL18_ODT-OFF_HYST-OFF_HSIO_I
117N   SLVSE_8mA_SLEW-OFF_N_O   SLVSE_8mA_SLEW-OFF_N_HSIO_O
117P   SLVSE_8mA_SLEW-OFF_P_O   SLVSE_8mA_SLEW-OFF_P_HSIO_O
118N   LVSTL11D_C1_40ohm_SLEW-OFF_N_O   LVSTL11_C1_40ohm_SLEW-OFF_HSIO_O
118P   LVSTL11D_C1_40ohm_SLEW-OFF_P_O   LVSTL11_C1_40ohm_SLEW-OFF_HSIO_O
119N   LVSTL11D_C1_120ohm_SLEW-OFF_N_O   LVSTL11_C1_120ohm_SLEW-OFF_HSIO_O
119P   LVSTL11D_C1_120ohm_SLEW-OFF_P_O   LVSTL11_C1_120ohm_SLEW-OFF_HSIO_O
120N   LVSTL11D_C1_80ohm_SLEW-OFF_N_O   LVSTL11_C1_80ohm_SLEW-OFF_HSIO_O
120P   LVSTL11D_C1_80ohm_SLEW-OFF_P_O   LVSTL11_C1_80ohm_SLEW-OFF_HSIO_O
121N   LVSTL11D_C1_60ohm_SLEW-OFF_N_O   LVSTL11_C1_60ohm_SLEW-OFF_HSIO_O
121P   LVSTL11D_C1_60ohm_SLEW-OFF_P_O   LVSTL11_C1_60ohm_SLEW-OFF_HSIO_O
122N   LVSTL11D_C1_48ohm_SLEW-OFF_N_O   LVSTL11_C1_48ohm_SLEW-OFF_HSIO_O
122P   LVSTL11D_C1_48ohm_SLEW-OFF_P_O   LVSTL11_C1_48ohm_SLEW-OFF_HSIO_O
123N   LVSTL11D_C1_34ohm_SLEW-OFF_N_O   LVSTL11_C1_34ohm_SLEW-OFF_HSIO_O
123P   LVSTL11D_C1_34ohm_SLEW-OFF_P_O   LVSTL11_C1_34ohm_SLEW-OFF_HSIO_O
124N   LVSTL11D_ODT-OFF_HYST-OFF_N_I   LVSTL11_ODT-OFF_HYST-OFF_HSIO_I
124P   LVSTL11D_ODT-OFF_HYST-OFF_P_I   LVSTL11_ODT-OFF_HYST-OFF_HSIO_I
125N   LVSTL11D_ODT-60_HYST-OFF_N_I   LVSTL11_ODT-60_HYST-OFF_HSIO_I
125P   LVSTL11D_ODT-60_HYST-OFF_P_I   LVSTL11_ODT-60_HYST-OFF_HSIO_I
126N   LVSTL11D_ODT-120_HYST-OFF_N_I   LVSTL11_ODT-120_HYST-OFF_HSIO_I
126P   LVSTL11D_ODT-120_HYST-OFF_P_I   LVSTL11_ODT-120_HYST-OFF_HSIO_I
127N   LVSTL11D_ODT-80_HYST-OFF_N_I   LVSTL11_ODT-80_HYST-OFF_HSIO_I
127P   LVSTL11D_ODT-80_HYST-OFF_P_I   LVSTL11_ODT-80_HYST-OFF_HSIO_I
128N   LVSTL11D_ODT-48_HYST-OFF_N_I   LVSTL11_ODT-48_HYST-OFF_HSIO_I
128P   LVSTL11D_ODT-48_HYST-OFF_P_I   LVSTL11_ODT-48_HYST-OFF_HSIO_I
129N   LVSTL11D_ODT-40_HYST-OFF_N_I   LVSTL11_ODT-40_HYST-OFF_HSIO_I
129P   LVSTL11D_ODT-40_HYST-OFF_P_I   LVSTL11_ODT-40_HYST-OFF_HSIO_I
130N   LVDS18_OD-OFF_HYST-OFF_VCML_N_I   LVDS18_OD-OFF_HYS-OFF_VCML_HSIO_I
130P   LVDS18_OD-OFF_HYST-OFF_VCML_P_I   LVDS18_OD-OFF_HYS-OFF_VCML_HSIO_I
131N   LVDS18_OD-OFF_HYST-OFF_VCMM_N_I   LVDS18_ODT-OFF_HYST-OFF_HSIO_I
131P   LVDS18_OD-OFF_HYST-OFF_VCMM_P_I   LVDS18_ODT-OFF_HYST-OFF_HSIO_I
132N   RSDS18_OD-OFF_HYST-OFF_VCML_N_I   RSDS18_OD-OFF_HYS-OFF_VCML_HSIO_I
132P   RSDS18_OD-OFF_HYST-OFF_VCML_P_I   RSDS18_OD-OFF_HYS-OFF_VCML_HSIO_I
133N   RSDS18_OD-OFF_HYST-OFF_VCMM_N_I   RSDS18_ODT-OFF_HYST-OFF_HSIO_I
133P   RSDS18_OD-OFF_HYST-OFF_VCMM_P_I   RSDS18_ODT-OFF_HYST-OFF_HSIO_I
134N   MINILVDS18_OD-OFF_HYST-OFF_VCML_N_I  MINILVDS18_OD-OFF_HYS-OFF_VCML_HSIO_I
134P   MINILVDS18_OD-OFF_HYST-OFF_VCML_P_I  MINILVDS18_OD-OFF_HYS-OFF_VCML_HSIO_I
135N   MINILVDS18_OD-OFF_HYST-OFF_VCMM_N_I  MINILVDS18_ODT-OFF_HYST-OFF_HSIO_I
135P   MINILVDS18_OD-OFF_HYST-OFF_VCMM_P_I  MINILVDS18_ODT-OFF_HYST-OFF_HSIO_I
136N   SUBLVDS18_OD-OFF_HYST-OFF_VCML_N_I   SUBLVDS18_OD-OFF_HYS-OFF_VCML_HSIO_I
136P   SUBLVDS18_OD-OFF_HYST-OFF_VCML_P_I   SUBLVDS18_OD-OFF_HYS-OFF_VCML_HSIO_I
137N   SUBLVDS18_OD-OFF_HYST-OFF_VCMM_N_I   SUBLVDS18_ODT-OFF_HYST-OFF_HSIO_I
137P   SUBLVDS18_OD-OFF_HYST-OFF_VCMM_P_I   SUBLVDS18_ODT-OFF_HYST-OFF_HSIO_I
138N   PPDS18_OD-OFF_HYST-OFF_VCML_N_I   PPDS18_OD-OFF_HYS-OFF_VCML_HSIO_I
138P   PPDS18_OD-OFF_HYST-OFF_VCML_P_I   PPDS18_OD-OFF_HYS-OFF_VCML_HSIO_I
139N   PPDS18_OD-OFF_HYST-OFF_VCMM_N_I   PPDS18_ODT-OFF_HYST-OFF_HSIO_I
139P   PPDS18_OD-OFF_HYST-OFF_VCMM_P_I   PPDS18_ODT-OFF_HYST-OFF_HSIO_I
140N   SLVS18_OD-OFF_HYST-OFF_VCML_N_I   SLVS18_OD-OFF_HYS-OFF_VCML_N_HSIO_I
140P   SLVS18_OD-OFF_HYST-OFF_VCML_P_I   SLVS18_OD-OFF_HYS-OFF_VCML_P_HSIO_I
141N   SLVS18_OD-OFF_HYST-OFF_VCMM_N_I   SLVS18_ODT-OFF_HYST-OFF_N_HSIO_I
141P   SLVS18_OD-OFF_HYST-OFF_VCMM_P_I   SLVS18_ODT-OFF_HYST-OFF_P_HSIO_I
142N   HCSL18_OD-OFF_HYST-OFF_VCML_N_I   HCSL18_OD-OFF_HYS-OFF_VCML_HSIO_I
142P   HCSL18_OD-OFF_HYST-OFF_VCML_P_I   HCSL18_OD-OFF_HYS-OFF_VCML_HSIO_I
143N   HCSL18_OD-OFF_HYST-OFF_VCMM_N_I   HCSL18_ODT-OFF_HYST-OFF_HSIO_I
143P   HCSL18_OD-OFF_HYST-OFF_VCMM_P_I   HCSL18_ODT-OFF_HYST-OFF_HSIO_I
144N   HSTL12D_18_ODT-OFF_HYST-OFF_N_I   HSTL12_18_ODT-OFF_HYST-OFF_HSIO_I
144P   HSTL12D_18_ODT-OFF_HYST-OFF_P_I   HSTL12_18_ODT-OFF_HYST-OFF_HSIO_I
145N   HSTL12D_15_ODT-OFF_HYST-OFF_N_I   HSTL12_15_ODT-OFF_HYST-OFF_HSIO_I
145P   HSTL12D_15_ODT-OFF_HYST-OFF_P_I   HSTL12_15_ODT-OFF_HYST-OFF_HSIO_I
146N   HSTL12D_135_ODT-OFF_HYST-OFF_N_I   HSTL12_135_ODT-OFF_HYST-OFF_HSIO_I
146P   HSTL12D_135_ODT-OFF_HYST-OFF_P_I   HSTL12_135_ODT-OFF_HYST-OFF_HSIO_I
147N   HSTL135D_18_ODT-OFF_HYST-OFF_N_I   HSTL135_18_ODT-OFF_HYST-OFF_HSIO_I
147P   HSTL135D_18_ODT-OFF_HYST-OFF_P_I   HSTL135_18_ODT-OFF_HYST-OFF_HSIO_I
148N   HSTL135D_15_ODT-OFF_HYST-OFF_N_I   HSTL135_15_ODT-OFF_HYST-OFF_HSIO_I
148P   HSTL135D_15_ODT-OFF_HYST-OFF_P_I   HSTL135_15_ODT-OFF_HYST-OFF_HSIO_I
149N   HSTL15D_18_ODT-OFF_HYST-OFF_N_I   HSTL15_18_ODT-OFF_HYST-OFF_HSIO_I
149P   HSTL15D_18_ODT-OFF_HYST-OFF_P_I   HSTL15_18_ODT-OFF_HYST-OFF_HSIO_I
150N   HSUL12D_18_ODT-OFF_HYST-OFF_N_I   HSUL12_18_ODT-OFF_HYST-OFF_HSIO_I
150P   HSUL12D_18_ODT-OFF_HYST-OFF_P_I   HSUL12_18_ODT-OFF_HYST-OFF_HSIO_I
151N   HSUL12D_15_ODT-OFF_HYST-OFF_N_I   HSUL12_15_ODT-OFF_HYST-OFF_HSIO_I
151P   HSUL12D_15_ODT-OFF_HYST-OFF_P_I   HSUL12_15_ODT-OFF_HYST-OFF_HSIO_I
152N   HSUL12D_135_ODT-OFF_HYST-OFF_N_I   HSUL12_135_ODT-OFF_HYST-OFF_HSIO_I
152P   HSUL12D_135_ODT-OFF_HYST-OFF_P_I   HSUL12_135_ODT-OFF_HYST-OFF_HSIO_I
153N   HSUL12D_18_ODT-60_HYST-OFF_N_I   HSUL12_18_ODT-60_HYST-OFF_HSIO_I
153P   HSUL12D_18_ODT-60_HYST-OFF_P_I   HSUL12_18_ODT-60_HYST-OFF_HSIO_I
154N   HSUL12D_15_ODT-60_HYST-OFF_N_I   HSUL12_15_ODT-60_HYST-OFF_HSIO_I
154P   HSUL12D_15_ODT-60_HYST-OFF_P_I   HSUL12_15_ODT-60_HYST-OFF_HSIO_I
155N   HSUL12D_135_ODT-60_HYST-OFF_N_I   HSUL12_135_ODT-60_HYST-OFF_HSIO_I
155P   HSUL12D_135_ODT-60_HYST-OFF_P_I   HSUL12_135_ODT-60_HYST-OFF_HSIO_I
156N   HSUL12D_18_ODT-240_HYST-OFF_N_I   HSUL12_18_ODT-240_HYST-OFF_HSIO_I
156P   HSUL12D_18_ODT-240_HYST-OFF_P_I   HSUL12_18_ODT-240_HYST-OFF_HSIO_I
157N   HSUL12D_15_ODT-240_HYST-OFF_N_I   HSUL12_15_ODT-240_HYST-OFF_HSIO_I
157P   HSUL12D_15_ODT-240_HYST-OFF_P_I   HSUL12_15_ODT-240_HYST-OFF_HSIO_I
158N   HSUL12D_135_ODT-240_HYST-OFF_N_I   HSUL12_135_ODT-240_HYST-OFF_HSIO_I
158P   HSUL12D_135_ODT-240_HYST-OFF_P_I   HSUL12_135_ODT-240_HYST-OFF_HSIO_I
159N   HSUL12D_18_ODT-120_HYST-OFF_N_I   HSUL12_18_ODT-120_HYST-OFF_HSIO_I
159P   HSUL12D_18_ODT-120_HYST-OFF_P_I   HSUL12_18_ODT-120_HYST-OFF_HSIO_I
160N   HSUL12D_15_ODT-120_HYST-OFF_N_I   HSUL12_15_ODT-120_HYST-OFF_HSIO_I
160P   HSUL12D_15_ODT-120_HYST-OFF_P_I   HSUL12_15_ODT-120_HYST-OFF_HSIO_I
161N   HSUL12D_135_ODT-120_HYST-OFF_N_I   HSUL12_135_ODT-120_HYST-OFF_HSIO_I
161P   HSUL12D_135_ODT-120_HYST-OFF_P_I   HSUL12_135_ODT-120_HYST-OFF_HSIO_I
162N   POD12D_18_ODT-OFF_HYST-OFF_N_I   POD12_18_ODT-OFF_HYST-OFF_HSIO_I
162P   POD12D_18_ODT-OFF_HYST-OFF_P_I   POD12_18_ODT-OFF_HYST-OFF_HSIO_I
163N   POD12D_15_ODT-OFF_HYST-OFF_N_I   POD12_15_ODT-OFF_HYST-OFF_HSIO_I
163P   POD12D_15_ODT-OFF_HYST-OFF_P_I   POD12_15_ODT-OFF_HYST-OFF_HSIO_I
164N   POD12D_135_ODT-OFF_HYST-OFF_N_I   POD12_135_ODT-OFF_HYST-OFF_HSIO_I
164P   POD12D_135_ODT-OFF_HYST-OFF_P_I   POD12_135_ODT-OFF_HYST-OFF_HSIO_I
165N   SSTL135D_18_ODT-OFF_HYST-OFF_N_I   SSTL135_18_ODT-OFF_HYST-OFF_HSIO_I
165P   SSTL135D_18_ODT-OFF_HYST-OFF_P_I   SSTL135_18_ODT-OFF_HYST-OFF_HSIO_I
166N   SSTL135D_15_ODT-OFF_HYST-OFF_N_I   SSTL135_15_ODT-OFF_HYST-OFF_HSIO_I
166P   SSTL135D_15_ODT-OFF_HYST-OFF_P_I   SSTL135_15_ODT-OFF_HYST-OFF_HSIO_I
167N   SSTL15D_18_ODT-OFF_HYST-OFF_N_I   SSTL15_18_ODT-OFF_HYST-OFF_HSIO_I
167P   SSTL15D_18_ODT-OFF_HYST-OFF_P_I   SSTL15_18_ODT-OFF_HYST-OFF_HSIO_I
168   VDDI   POWER
169   VSS   GND
[Pin Mapping]   pulldown_ref   pullup_ref   gnd_clamp_ref   power_clamp_ref   ext_ref
1N   VSS   VDDI   VSS   VDDI
1P   VSS   VDDI   VSS   VDDI
2N   VSS   VDDI   VSS   VDDI
2P   VSS   VDDI   VSS   VDDI
3N   VSS   VDDI   VSS   VDDI
3P   VSS   VDDI   VSS   VDDI
4N   VSS   VDDI   VSS   VDDI
4P   VSS   VDDI   VSS   VDDI
5N   VSS   VDDI   VSS   VDDI
5P   VSS   VDDI   VSS   VDDI
6N   VSS   VDDI   VSS   VDDI
6P   VSS   VDDI   VSS   VDDI
7N   VSS   VDDI   VSS   VDDI
7P   VSS   VDDI   VSS   VDDI
8N   VSS   VDDI   VSS   VDDI
8P   VSS   VDDI   VSS   VDDI
9N   VSS   VDDI   VSS   VDDI
9P   VSS   VDDI   VSS   VDDI
10N   VSS   VDDI   VSS   VDDI
10P   VSS   VDDI   VSS   VDDI
11N   VSS   VDDI   VSS   VDDI
11P   VSS   VDDI   VSS   VDDI
12N   VSS   VDDI   VSS   VDDI
12P   VSS   VDDI   VSS   VDDI
13N   VSS   VDDI   VSS   VDDI
13P   VSS   VDDI   VSS   VDDI
14N   VSS   VDDI   VSS   VDDI
14P   VSS   VDDI   VSS   VDDI
15N   VSS   VDDI   VSS   VDDI
15P   VSS   VDDI   VSS   VDDI
16N   VSS   VDDI   VSS   VDDI
16P   VSS   VDDI   VSS   VDDI
17N   VSS   VDDI   VSS   VDDI
17P   VSS   VDDI   VSS   VDDI
18N   VSS   VDDI   VSS   VDDI
18P   VSS   VDDI   VSS   VDDI
19N   VSS   VDDI   VSS   VDDI
19P   VSS   VDDI   VSS   VDDI
20N   VSS   VDDI   VSS   VDDI
20P   VSS   VDDI   VSS   VDDI
21N   VSS   VDDI   VSS   VDDI
21P   VSS   VDDI   VSS   VDDI
22N   VSS   VDDI   VSS   VDDI
22P   VSS   VDDI   VSS   VDDI
23N   VSS   VDDI   VSS   VDDI
23P   VSS   VDDI   VSS   VDDI
24N   VSS   VDDI   VSS   VDDI
24P   VSS   VDDI   VSS   VDDI
25N   VSS   VDDI   VSS   VDDI
25P   VSS   VDDI   VSS   VDDI
26N   VSS   VDDI   VSS   VDDI
26P   VSS   VDDI   VSS   VDDI
27N   VSS   VDDI   VSS   VDDI
27P   VSS   VDDI   VSS   VDDI
28N   VSS   VDDI   VSS   VDDI
28P   VSS   VDDI   VSS   VDDI
29N   VSS   VDDI   VSS   VDDI
29P   VSS   VDDI   VSS   VDDI
30N   VSS   VDDI   VSS   VDDI
30P   VSS   VDDI   VSS   VDDI
31N   VSS   VDDI   VSS   VDDI
31P   VSS   VDDI   VSS   VDDI
32N   VSS   VDDI   VSS   VDDI
32P   VSS   VDDI   VSS   VDDI
33N   VSS   VDDI   VSS   VDDI
33P   VSS   VDDI   VSS   VDDI
34N   VSS   VDDI   VSS   VDDI
34P   VSS   VDDI   VSS   VDDI
35N   VSS   VDDI   VSS   VDDI
35P   VSS   VDDI   VSS   VDDI
36N   VSS   VDDI   VSS   VDDI
36P   VSS   VDDI   VSS   VDDI
37N   VSS   VDDI   VSS   VDDI
37P   VSS   VDDI   VSS   VDDI
38N   VSS   VDDI   VSS   VDDI
38P   VSS   VDDI   VSS   VDDI
39N   VSS   VDDI   VSS   VDDI
39P   VSS   VDDI   VSS   VDDI
40N   VSS   VDDI   VSS   VDDI
40P   VSS   VDDI   VSS   VDDI
41N   VSS   VDDI   VSS   VDDI
41P   VSS   VDDI   VSS   VDDI
42N   VSS   VDDI   VSS   VDDI
42P   VSS   VDDI   VSS   VDDI
43N   VSS   VDDI   VSS   VDDI
43P   VSS   VDDI   VSS   VDDI
44N   VSS   VDDI   VSS   VDDI
44P   VSS   VDDI   VSS   VDDI
45N   VSS   VDDI   VSS   VDDI
45P   VSS   VDDI   VSS   VDDI
46N   VSS   VDDI   VSS   VDDI
46P   VSS   VDDI   VSS   VDDI
47N   VSS   VDDI   VSS   VDDI
47P   VSS   VDDI   VSS   VDDI
48N   VSS   VDDI   VSS   VDDI
48P   VSS   VDDI   VSS   VDDI
49N   VSS   VDDI   VSS   VDDI
49P   VSS   VDDI   VSS   VDDI
50N   VSS   VDDI   VSS   VDDI
50P   VSS   VDDI   VSS   VDDI
51N   VSS   VDDI   VSS   VDDI
51P   VSS   VDDI   VSS   VDDI
52N   VSS   VDDI   VSS   VDDI
52P   VSS   VDDI   VSS   VDDI
53N   VSS   VDDI   VSS   VDDI
53P   VSS   VDDI   VSS   VDDI
54N   VSS   VDDI   VSS   VDDI
54P   VSS   VDDI   VSS   VDDI
55N   VSS   VDDI   VSS   VDDI
55P   VSS   VDDI   VSS   VDDI
56N   VSS   VDDI   VSS   VDDI
56P   VSS   VDDI   VSS   VDDI
57N   VSS   VDDI   VSS   VDDI
57P   VSS   VDDI   VSS   VDDI
58N   VSS   VDDI   VSS   VDDI
58P   VSS   VDDI   VSS   VDDI
59N   VSS   VDDI   VSS   VDDI
59P   VSS   VDDI   VSS   VDDI
60N   VSS   VDDI   VSS   VDDI
60P   VSS   VDDI   VSS   VDDI
61N   VSS   VDDI   VSS   VDDI
61P   VSS   VDDI   VSS   VDDI
62N   VSS   VDDI   VSS   VDDI
62P   VSS   VDDI   VSS   VDDI
63N   VSS   VDDI   VSS   VDDI
63P   VSS   VDDI   VSS   VDDI
64N   VSS   VDDI   VSS   VDDI
64P   VSS   VDDI   VSS   VDDI
65N   VSS   VDDI   VSS   VDDI
65P   VSS   VDDI   VSS   VDDI
66N   VSS   VDDI   VSS   VDDI
66P   VSS   VDDI   VSS   VDDI
67N   VSS   VDDI   VSS   VDDI
67P   VSS   VDDI   VSS   VDDI
68N   VSS   VDDI   VSS   VDDI
68P   VSS   VDDI   VSS   VDDI
69N   VSS   VDDI   VSS   VDDI
69P   VSS   VDDI   VSS   VDDI
70N   VSS   VDDI   VSS   VDDI
70P   VSS   VDDI   VSS   VDDI
71N   VSS   VDDI   VSS   VDDI
71P   VSS   VDDI   VSS   VDDI
72N   VSS   VDDI   VSS   VDDI
72P   VSS   VDDI   VSS   VDDI
73N   VSS   VDDI   VSS   VDDI
73P   VSS   VDDI   VSS   VDDI
74N   VSS   VDDI   VSS   VDDI
74P   VSS   VDDI   VSS   VDDI
75N   VSS   VDDI   VSS   VDDI
75P   VSS   VDDI   VSS   VDDI
76N   VSS   VDDI   VSS   VDDI
76P   VSS   VDDI   VSS   VDDI
77N   VSS   VDDI   VSS   VDDI
77P   VSS   VDDI   VSS   VDDI
78N   VSS   VDDI   VSS   VDDI
78P   VSS   VDDI   VSS   VDDI
79N   VSS   VDDI   VSS   VDDI
79P   VSS   VDDI   VSS   VDDI
80N   VSS   VDDI   VSS   VDDI
80P   VSS   VDDI   VSS   VDDI
81N   VSS   VDDI   VSS   VDDI
81P   VSS   VDDI   VSS   VDDI
82N   VSS   VDDI   VSS   VDDI
82P   VSS   VDDI   VSS   VDDI
83N   VSS   VDDI   VSS   VDDI
83P   VSS   VDDI   VSS   VDDI
84N   VSS   VDDI   VSS   VDDI
84P   VSS   VDDI   VSS   VDDI
85N   VSS   VDDI   VSS   VDDI
85P   VSS   VDDI   VSS   VDDI
86N   VSS   VDDI   VSS   VDDI
86P   VSS   VDDI   VSS   VDDI
87N   VSS   VDDI   VSS   VDDI
87P   VSS   VDDI   VSS   VDDI
88N   VSS   VDDI   VSS   VDDI
88P   VSS   VDDI   VSS   VDDI
89N   VSS   VDDI   VSS   VDDI
89P   VSS   VDDI   VSS   VDDI
90N   VSS   VDDI   VSS   VDDI
90P   VSS   VDDI   VSS   VDDI
91N   VSS   VDDI   VSS   VDDI
91P   VSS   VDDI   VSS   VDDI
92N   VSS   VDDI   VSS   VDDI
92P   VSS   VDDI   VSS   VDDI
93N   VSS   VDDI   VSS   VDDI
93P   VSS   VDDI   VSS   VDDI
94N   VSS   VDDI   VSS   VDDI
94P   VSS   VDDI   VSS   VDDI
95N   VSS   VDDI   VSS   VDDI
95P   VSS   VDDI   VSS   VDDI
96N   VSS   VDDI   VSS   VDDI
96P   VSS   VDDI   VSS   VDDI
97N   VSS   VDDI   VSS   VDDI
97P   VSS   VDDI   VSS   VDDI
98N   VSS   VDDI   VSS   VDDI
98P   VSS   VDDI   VSS   VDDI
99N   VSS   VDDI   VSS   VDDI
99P   VSS   VDDI   VSS   VDDI
100N   VSS   VDDI   VSS   VDDI
100P   VSS   VDDI   VSS   VDDI
101N   VSS   VDDI   VSS   VDDI
101P   VSS   VDDI   VSS   VDDI
102N   VSS   VDDI   VSS   VDDI
102P   VSS   VDDI   VSS   VDDI
103N   VSS   VDDI   VSS   VDDI
103P   VSS   VDDI   VSS   VDDI
104N   VSS   VDDI   VSS   VDDI
104P   VSS   VDDI   VSS   VDDI
105N   VSS   VDDI   VSS   VDDI
105P   VSS   VDDI   VSS   VDDI
106N   VSS   VDDI   VSS   VDDI
106P   VSS   VDDI   VSS   VDDI
107N   VSS   VDDI   VSS   VDDI
107P   VSS   VDDI   VSS   VDDI
108N   VSS   VDDI   VSS   VDDI
108P   VSS   VDDI   VSS   VDDI
109N   VSS   VDDI   VSS   VDDI
109P   VSS   VDDI   VSS   VDDI
110N   VSS   VDDI   VSS   VDDI
110P   VSS   VDDI   VSS   VDDI
111N   VSS   VDDI   VSS   VDDI
111P   VSS   VDDI   VSS   VDDI
112N   VSS   VDDI   VSS   VDDI
112P   VSS   VDDI   VSS   VDDI
113N   VSS   VDDI   VSS   VDDI
113P   VSS   VDDI   VSS   VDDI
114N   VSS   VDDI   VSS   VDDI
114P   VSS   VDDI   VSS   VDDI
115N   VSS   VDDI   VSS   VDDI
115P   VSS   VDDI   VSS   VDDI
116N   VSS   VDDI   VSS   VDDI
116P   VSS   VDDI   VSS   VDDI
117N   VSS   VDDI   VSS   VDDI
117P   VSS   VDDI   VSS   VDDI
118N   VSS   VDDI   VSS   VDDI
118P   VSS   VDDI   VSS   VDDI
119N   VSS   VDDI   VSS   VDDI
119P   VSS   VDDI   VSS   VDDI
120N   VSS   VDDI   VSS   VDDI
120P   VSS   VDDI   VSS   VDDI
121N   VSS   VDDI   VSS   VDDI
121P   VSS   VDDI   VSS   VDDI
122N   VSS   VDDI   VSS   VDDI
122P   VSS   VDDI   VSS   VDDI
123N   VSS   VDDI   VSS   VDDI
123P   VSS   VDDI   VSS   VDDI
124N   VSS   VDDI   VSS   VDDI
124P   VSS   VDDI   VSS   VDDI
125N   VSS   VDDI   VSS   VDDI
125P   VSS   VDDI   VSS   VDDI
126N   VSS   VDDI   VSS   VDDI
126P   VSS   VDDI   VSS   VDDI
127N   VSS   VDDI   VSS   VDDI
127P   VSS   VDDI   VSS   VDDI
128N   VSS   VDDI   VSS   VDDI
128P   VSS   VDDI   VSS   VDDI
129N   VSS   VDDI   VSS   VDDI
129P   VSS   VDDI   VSS   VDDI
130N   VSS   VDDI   VSS   VDDI
130P   VSS   VDDI   VSS   VDDI
131N   VSS   VDDI   VSS   VDDI
131P   VSS   VDDI   VSS   VDDI
132N   VSS   VDDI   VSS   VDDI
132P   VSS   VDDI   VSS   VDDI
133N   VSS   VDDI   VSS   VDDI
133P   VSS   VDDI   VSS   VDDI
134N   VSS   VDDI   VSS   VDDI
134P   VSS   VDDI   VSS   VDDI
135N   VSS   VDDI   VSS   VDDI
135P   VSS   VDDI   VSS   VDDI
136N   VSS   VDDI   VSS   VDDI
136P   VSS   VDDI   VSS   VDDI
137N   VSS   VDDI   VSS   VDDI
137P   VSS   VDDI   VSS   VDDI
138N   VSS   VDDI   VSS   VDDI
138P   VSS   VDDI   VSS   VDDI
139N   VSS   VDDI   VSS   VDDI
139P   VSS   VDDI   VSS   VDDI
140N   VSS   VDDI   VSS   VDDI
140P   VSS   VDDI   VSS   VDDI
141N   VSS   VDDI   VSS   VDDI
141P   VSS   VDDI   VSS   VDDI
142N   VSS   VDDI   VSS   VDDI
142P   VSS   VDDI   VSS   VDDI
143N   VSS   VDDI   VSS   VDDI
143P   VSS   VDDI   VSS   VDDI
144N   VSS   VDDI   VSS   VDDI
144P   VSS   VDDI   VSS   VDDI
145N   VSS   VDDI   VSS   VDDI
145P   VSS   VDDI   VSS   VDDI
146N   VSS   VDDI   VSS   VDDI
146P   VSS   VDDI   VSS   VDDI
147N   VSS   VDDI   VSS   VDDI
147P   VSS   VDDI   VSS   VDDI
148N   VSS   VDDI   VSS   VDDI
148P   VSS   VDDI   VSS   VDDI
149N   VSS   VDDI   VSS   VDDI
149P   VSS   VDDI   VSS   VDDI
150N   VSS   VDDI   VSS   VDDI
150P   VSS   VDDI   VSS   VDDI
151N   VSS   VDDI   VSS   VDDI
151P   VSS   VDDI   VSS   VDDI
152N   VSS   VDDI   VSS   VDDI
152P   VSS   VDDI   VSS   VDDI
153N   VSS   VDDI   VSS   VDDI
153P   VSS   VDDI   VSS   VDDI
154N   VSS   VDDI   VSS   VDDI
154P   VSS   VDDI   VSS   VDDI
155N   VSS   VDDI   VSS   VDDI
155P   VSS   VDDI   VSS   VDDI
156N   VSS   VDDI   VSS   VDDI
156P   VSS   VDDI   VSS   VDDI
157N   VSS   VDDI   VSS   VDDI
157P   VSS   VDDI   VSS   VDDI
158N   VSS   VDDI   VSS   VDDI
158P   VSS   VDDI   VSS   VDDI
159N   VSS   VDDI   VSS   VDDI
159P   VSS   VDDI   VSS   VDDI
160N   VSS   VDDI   VSS   VDDI
160P   VSS   VDDI   VSS   VDDI
161N   VSS   VDDI   VSS   VDDI
161P   VSS   VDDI   VSS   VDDI
162N   VSS   VDDI   VSS   VDDI
162P   VSS   VDDI   VSS   VDDI
163N   VSS   VDDI   VSS   VDDI
163P   VSS   VDDI   VSS   VDDI
164N   VSS   VDDI   VSS   VDDI
164P   VSS   VDDI   VSS   VDDI
165N   VSS   VDDI   VSS   VDDI
165P   VSS   VDDI   VSS   VDDI
166N   VSS   VDDI   VSS   VDDI
166P   VSS   VDDI   VSS   VDDI
167N   VSS   VDDI   VSS   VDDI
167P   VSS   VDDI   VSS   VDDI
168   NC   VDDI
169   VSS   NC
[Diff Pin]   inv_pin   vdiff   tdelay_typ   tdelay_min   tdelay_max
1P   1N   100mV   0   0   0
2P   2N   100mV   0   0   0
3P   3N   100mV   0   0   0
4P   4N   100mV   0   0   0
5P   5N   100mV   0   0   0
6P   6N   100mV   0   0   0
7P   7N   100mV   0   0   0
8P   8N   100mV   0   0   0
9P   9N   100mV   0   0   0
10P   10N   100mV   0   0   0
11P   11N   100mV   0   0   0
12P   12N   100mV   0   0   0
13P   13N   100mV   0   0   0
14P   14N   100mV   0   0   0
15P   15N   100mV   0   0   0
16P   16N   100mV   0   0   0
17P   17N   100mV   0   0   0
18P   18N   100mV   0   0   0
19P   19N   100mV   0   0   0
20P   20N   100mV   0   0   0
21P   21N   100mV   0   0   0
22P   22N   100mV   0   0   0
23P   23N   100mV   0   0   0
24P   24N   100mV   0   0   0
25P   25N   100mV   0   0   0
26P   26N   100mV   0   0   0
27P   27N   100mV   0   0   0
28P   28N   100mV   0   0   0
29P   29N   100mV   0   0   0
30P   30N   100mV   0   0   0
31P   31N   100mV   0   0   0
32P   32N   100mV   0   0   0
33P   33N   100mV   0   0   0
34P   34N   100mV   0   0   0
35P   35N   100mV   0   0   0
36P   36N   100mV   0   0   0
37P   37N   100mV   0   0   0
38P   38N   100mV   0   0   0
39P   39N   100mV   0   0   0
40P   40N   100mV   0   0   0
41P   41N   100mV   0   0   0
42P   42N   100mV   0   0   0
43P   43N   100mV   0   0   0
44P   44N   100mV   0   0   0
45P   45N   100mV   0   0   0
46P   46N   100mV   0   0   0
47P   47N   100mV   0   0   0
48P   48N   100mV   0   0   0
49P   49N   100mV   0   0   0
50P   50N   100mV   0   0   0
51P   51N   100mV   0   0   0
52P   52N   100mV   0   0   0
53P   53N   100mV   0   0   0
54P   54N   100mV   0   0   0
55P   55N   100mV   0   0   0
56P   56N   100mV   0   0   0
57P   57N   100mV   0   0   0
58P   58N   100mV   0   0   0
59P   59N   100mV   0   0   0
60P   60N   100mV   0   0   0
61P   61N   100mV   0   0   0
62P   62N   100mV   0   0   0
63P   63N   100mV   0   0   0
64P   64N   100mV   0   0   0
65P   65N   100mV   0   0   0
66P   66N   100mV   0   0   0
67P   67N   100mV   0   0   0
68P   68N   100mV   0   0   0
69P   69N   100mV   0   0   0
70P   70N   100mV   0   0   0
71P   71N   100mV   0   0   0
72P   72N   100mV   0   0   0
73P   73N   100mV   0   0   0
74P   74N   100mV   0   0   0
75P   75N   100mV   0   0   0
76P   76N   100mV   0   0   0
77P   77N   100mV   0   0   0
78P   78N   100mV   0   0   0
79P   79N   100mV   0   0   0
80P   80N   100mV   0   0   0
81P   81N   100mV   0   0   0
82P   82N   100mV   0   0   0
83P   83N   100mV   0   0   0
84P   84N   100mV   0   0   0
85P   85N   100mV   0   0   0
86P   86N   100mV   0   0   0
87P   87N   100mV   0   0   0
88P   88N   100mV   0   0   0
89P   89N   100mV   0   0   0
90P   90N   100mV   0   0   0
91P   91N   100mV   0   0   0
92P   92N   100mV   0   0   0
93P   93N   100mV   0   0   0
94P   94N   100mV   0   0   0
95P   95N   100mV   0   0   0
96P   96N   100mV   0   0   0
97P   97N   100mV   0   0   0
98P   98N   100mV   0   0   0
99P   99N   100mV   0   0   0
100P   100N   100mV   0   0   0
101P   101N   100mV   0   0   0
102P   102N   100mV   0   0   0
103P   103N   100mV   0   0   0
104P   104N   100mV   0   0   0
105P   105N   100mV   0   0   0
106P   106N   100mV   0   0   0
107P   107N   100mV   0   0   0
108P   108N   100mV   0   0   0
109P   109N   100mV   0   0   0
110P   110N   100mV   0   0   0
111P   111N   100mV   0   0   0
112P   112N   100mV   0   0   0
113P   113N   100mV   0   0   0
114P   114N   100mV   0   0   0
115P   115N   100mV   0   0   0
116P   116N   100mV   0   0   0
117P   117N   100mV   0   0   0
118P   118N   100mV   0   0   0
119P   119N   100mV   0   0   0
120P   120N   100mV   0   0   0
121P   121N   100mV   0   0   0
122P   122N   100mV   0   0   0
123P   123N   100mV   0   0   0
124P   124N   100mV   0   0   0
125P   125N   100mV   0   0   0
126P   126N   100mV   0   0   0
127P   127N   100mV   0   0   0
128P   128N   100mV   0   0   0
129P   129N   100mV   0   0   0
130P   130N   100mV   0   0   0
131P   131N   100mV   0   0   0
132P   132N   100mV   0   0   0
133P   133N   100mV   0   0   0
134P   134N   100mV   0   0   0
135P   135N   100mV   0   0   0
136P   136N   100mV   0   0   0
137P   137N   100mV   0   0   0
138P   138N   100mV   0   0   0
139P   139N   100mV   0   0   0
140P   140N   100mV   0   0   0
141P   141N   100mV   0   0   0
142P   142N   100mV   0   0   0
143P   143N   100mV   0   0   0
144P   144N   100mV   0   0   0
145P   145N   100mV   0   0   0
146P   146N   100mV   0   0   0
147P   147N   100mV   0   0   0
148P   148N   100mV   0   0   0
149P   149N   100mV   0   0   0
150P   150N   100mV   0   0   0
151P   151N   100mV   0   0   0
152P   152N   100mV   0   0   0
153P   153N   100mV   0   0   0
154P   154N   100mV   0   0   0
155P   155N   100mV   0   0   0
156P   156N   100mV   0   0   0
157P   157N   100mV   0   0   0
158P   158N   100mV   0   0   0
159P   159N   100mV   0   0   0
160P   160N   100mV   0   0   0
161P   161N   100mV   0   0   0
162P   162N   100mV   0   0   0
163P   163N   100mV   0   0   0
164P   164N   100mV   0   0   0
165P   165N   100mV   0   0   0
166P   166N   100mV   0   0   0
167P   167N   100mV   0   0   0
| Models and submodels in the file (163): LVCMOS18_8mA_SLEW-OFF_HSIO_O (Output), LVCMOS18_2mA_SLEW-OFF_HSIO_O (Output), LVCMOS18_4mA_SLEW-OFF_HSIO_O (Output), LVCMOS18_6mA_SLEW-OFF_HSIO_O (Output), LVCMOS18_10mA_SLEW-OFF_HSIO_O (Output), LVCMOS18_12mA_SLEW-OFF_HSIO_O (Output), LVCMOS15_8mA_SLEW-OFF_HSIO_O (Output), LVCMOS15_2mA_SLEW-OFF_HSIO_O (Output), LVCMOS15_4mA_SLEW-OFF_HSIO_O (Output), LVCMOS15_6mA_SLEW-OFF_HSIO_O (Output), LVCMOS15_10mA_SLEW-OFF_HSIO_O (Output), LVCMOS12_8mA_SLEW-OFF_HSIO_O (Output), LVCMOS12_2mA_SLEW-OFF_HSIO_O (Output), LVCMOS12_4mA_SLEW-OFF_HSIO_O (Output), LVCMOS12_6mA_SLEW-OFF_HSIO_O (Output), LVCMOS12_10mA_SLEW-OFF_HSIO_O (Output), SSTL18_C1_60ohm_SLEW-OFF_HSIO_O (Output), SSTL18_C1_80ohm_SLEW-OFF_HSIO_O (Output), SSTL18_C1_48ohm_SLEW-OFF_HSIO_O (Output), SSTL18_C1_40ohm_SLEW-OFF_HSIO_O (Output), SSTL18_C2_40ohm_SLEW-OFF_HSIO_O (Output), SSTL18_C2_48ohm_SLEW-OFF_HSIO_O (Output), SSTL18_C2_34ohm_SLEW-OFF_HSIO_O (Output), SSTL18_C2_30ohm_SLEW-OFF_HSIO_O (Output), SSTL15_C1_40ohm_SLEW-OFF_HSIO_O (Output), SSTL15_C1_48ohm_SLEW-OFF_HSIO_O (Output), SSTL15_C2_34ohm_SLEW-OFF_HSIO_O (Output), SSTL15_C2_30ohm_SLEW-OFF_HSIO_O (Output), SSTL15_C2_27ohm_SLEW-OFF_HSIO_O (Output), SSTL135_C1_40ohm_SLEW-OFF_HSIO_O (Output), SSTL135_C1_48ohm_SLEW-OFF_HSIO_O (Output), SSTL135_C2_34ohm_SLEW-OFF_HSIO_O (Output), SSTL135_C2_30ohm_SLEW-OFF_HSIO_O (Output), SSTL135_C2_27ohm_SLEW-OFF_HSIO_O (Output), HSUL18_C1_55ohm_SLEW-OFF_HSIO_O (Output), HSUL18_C1_60ohm_SLEW-OFF_HSIO_O (Output), HSUL18_C1_40ohm_SLEW-OFF_HSIO_O (Output), HSUL18_C1_34ohm_SLEW-OFF_HSIO_O (Output), HSUL18_C2_25ohm_SLEW-OFF_HSIO_O (Output), HSUL18_C2_30ohm_SLEW-OFF_HSIO_O (Output), HSUL18_C2_27ohm_SLEW-OFF_HSIO_O (Output), HSUL18_C2_22ohm_SLEW-OFF_HSIO_O (Output), HSTL15_C1_50ohm_SLEW-OFF_HSIO_O (Output), HSTL15_C1_60ohm_SLEW-OFF_HSIO_O (Output), HSTL15_C1_40ohm_SLEW-OFF_HSIO_O (Output), HSTL15_C1_34ohm_SLEW-OFF_HSIO_O (Output), HSTL15_C2_25ohm_SLEW-OFF_HSIO_O (Output), HSTL15_C2_30ohm_SLEW-OFF_HSIO_O (Output), HSTL15_C2_27ohm_SLEW-OFF_HSIO_O (Output), HSTL15_C2_22ohm_SLEW-OFF_HSIO_O (Output), HSTL135_C1_50ohm_SLEW-OFF_HSIO_O (Output), HSTL135_C1_60ohm_SLEW-OFF_HSIO_O (Output), HSTL135_C1_40ohm_SLEW-OFF_HSIO_O (Output), HSTL135_C1_34ohm_SLEW-OFF_HSIO_O (Output), HSTL135_C2_25ohm_SLEW-OFF_HSIO_O (Output), HSTL135_C2_30ohm_SLEW-OFF_HSIO_O (Output), HSTL135_C2_27ohm_SLEW-OFF_HSIO_O (Output), HSTL135_C2_22ohm_SLEW-OFF_HSIO_O (Output), HSUL12_40ohm_SLEW-OFF_HSIO_O (Output), HSUL12_120ohm_SLEW-OFF_HSIO_O (Output), HSUL12_80ohm_SLEW-OFF_HSIO_O (Output), HSUL12_60ohm_SLEW-OFF_HSIO_O (Output), HSUL12_48ohm_SLEW-OFF_HSIO_O (Output), HSUL12_34ohm_SLEW-OFF_HSIO_O (Output), POD12_C1_48ohm_SLEW-OFF_HSIO_O (Output), POD12_C1_60ohm_SLEW-OFF_HSIO_O (Output), POD12_C1_40ohm_SLEW-OFF_HSIO_O (Output), POD12_C2_34ohm_SLEW-OFF_HSIO_O (Output), POD12_C2_30ohm_SLEW-OFF_HSIO_O (Output), POD12_C2_27ohm_SLEW-OFF_HSIO_O (Output), HSTL12_C1_50ohm_SLEW-OFF_HSIO_O (Output), HSTL12_C2_25ohm_SLEW-OFF_HSIO_O (Output), SSTL18_ODT-OFF_HYST-OFF_HSIO_I (Input), SSTL18_ODT-50_HYST-OFF_HSIO_I (Input), SSTL18_ODT-150_HYST-OFF_HSIO_I (Input), SSTL18_ODT-75_HYST-OFF_HSIO_I (Input), SSTL15_ODT-OFF_HYST-OFF_HSIO_I (Input), SSTL15_ODT-60_HYST-OFF_HSIO_I (Input), SSTL15_ODT-120_HYST-OFF_HSIO_I (Input), SSTL15_ODT-40_HYST-OFF_HSIO_I (Input)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
